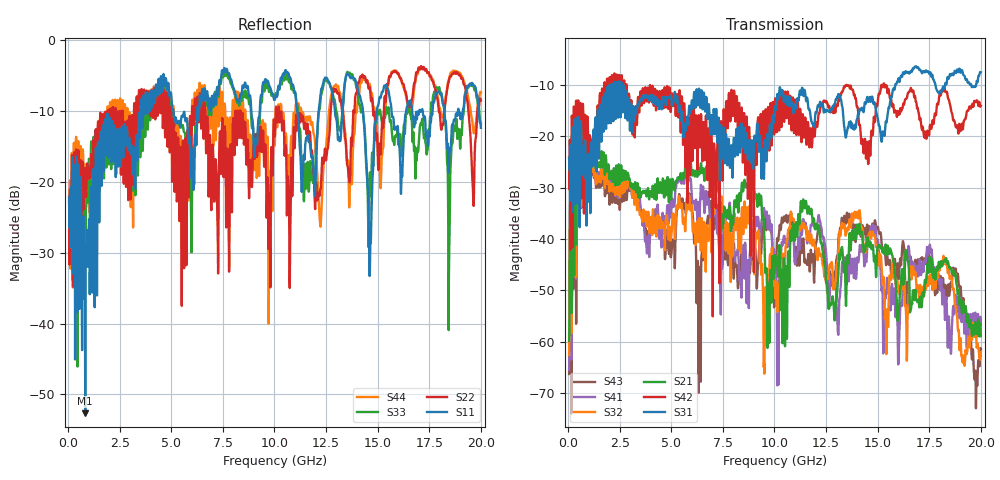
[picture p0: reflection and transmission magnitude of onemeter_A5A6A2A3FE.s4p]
! FILE: D:\iPass\iPassCable1005\iPassCable\SOLT_cal\onemeter_A5A6A2A3FE.s4p
# MHz S MA R 50.00
! FREQ  S11  S12  S13  S14
!  S21  S22  S23  S24
!  S31  S32  S33  S34
!  S41  S42  S43  S44
!  MAG  ANG  MAG  ANG  MAG  ANG  MAG  ANG
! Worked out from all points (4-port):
!   1996 points, 50 MHz to 20 GHz, reference 50 ohm
!   strongest paths, dB at 50 MHz, 5.04 GHz, 10.03 GHz, 15.02 GHz, 20 GHz:
!     S31: -24.2, -14.0, -14.3, -16.8, -7.6
!     S42: -24.1, -11.9, -12.9, -12.7, -14.1
!     S21: -59.8, -28.9, -43.4, -41.4, -58.9
!     S32: -62.6, -37.1, -51.5, -43.4, -62.0
!     S41: -65.4, -32.1, -48.3, -40.4, -56.6
!     S43: -66.2, -40.5, -45.3, -37.7, -61.3
!   lowest |S11| = -52.7 dB at 830 MHz (marker M1), VSWR 1.00, Z = 50.2 + j0.146 ohm
!   |S11| at or under -10 dB: start of sweep to 3.515 GHz; 5.107 GHz to 6.253 GHz (1.146 GHz wide, 20.2 % of centre); 11.1 GHz to 12.14 GHz (1.039 GHz wide, 8.94 % of centre)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
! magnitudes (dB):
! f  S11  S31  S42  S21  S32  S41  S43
! 50 MHz  -22.2  -24.2  -24.1  -59.8  -62.6  -65.4  -66.2
! 830 MHz  -52.7  -21.3  -15.9  -26.6  -29.2  -27.7  -29.5
! 4.57 GHz  -6.7  -12.4  -11.1  -29.4  -36.8  -35.3  -41.1
! 9.55 GHz  -5.5  -20.7  -15.8  -46.3  -49.9  -35.4  -36.1
! 13.83 GHz  -5.4  -18.1  -11.7  -39.9  -35.8  -46.5  -39.1
! 14.63 GHz  -30.8  -12.6  -23.4  -40.6  -38.6  -38.9  -38.0
! 20 GHz  -12.4  -7.6  -14.1  -58.9  -62.0  -56.6  -61.3
